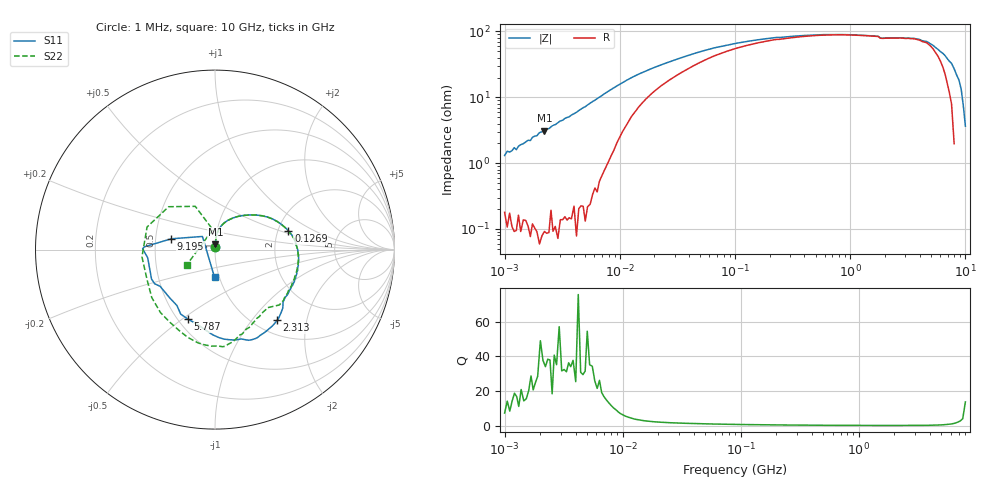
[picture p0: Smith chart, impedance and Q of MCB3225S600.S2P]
!Agilent Technologies,E5071C,MY46111244,A.11.31
!Date: Thu May 09 18:34:08 2019
!Data & Calibration Information:
!Freq	S11:SOLT2(ON)	S21:SOLT2(ON)	S12:SOLT2(ON)	S22:SOLT2(ON)
# Hz S dB R 50
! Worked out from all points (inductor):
!   201 points, 1 MHz to 10 GHz, reference 50 ohm
!   read as one part in series: L = 218 nH near 1.053 MHz
!   highest Q = 37.9 at 2.216 MHz (marker M1), where L = 224 nH
!   self-resonance near 9.967 GHz
!   S11 on the Smith chart (normalised r, x): 1 MHz: 1.00, +0.03; 126.9 MHz: 2.28, +0.58; 2.313 GHz: 1.24, -1.35; 5.787 GHz: 0.56, -0.53; 9.195 GHz: 0.60, +0.08; 10 GHz: 0.95, -0.30
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1000000  -37.49 83.9  -0.00 -0.7  -0.03 -0.7  -37.47 80.1
2216092  -30.49 85.7  -0.01 -1.8  -0.01 -1.9  -30.31 86.1
4810209  -23.33 84.3  -0.05 -4.0  -0.04 -4.1  -23.32 84.8
1.053043e7  -15.96 70.5  -0.37 -9.2  -0.37 -9.2  -15.98 70.6
2.206931e7  -11.82 48.3  -1.39 -13.5  -1.40 -13.5  -11.83 48.3
1.047129e8  -7.72 17.1  -4.08 -14.3  -4.08 -14.3  -7.72 17.0
1.269299e8  -7.49 14.3  -4.34 -13.8  -4.35 -13.8  -7.49 14.1
4.810209e8  -6.62 -4.6  -5.48 -12.4  -5.49 -12.4  -6.64 -5.2
1.380384e9  -6.51 -28.9  -5.72 -21.9  -5.71 -21.9  -6.54 -30.9
2.206931e9  -5.66 -47.1  -5.86 -34.0  -5.84 -34.0  -6.98 -56.3
2.312765e9  -5.61 -48.7  -5.93 -35.4  -5.94 -35.3  -6.97 -58.7
3.801894e9  -5.37 -69.7  -6.53 -51.0  -6.58 -50.9  -5.71 -78.2
4.83488e9  -6.19 -87.5  -6.55 -64.0  -6.54 -64.0  -5.39 -88.1
5.786901e9  -7.62 -111.0  -6.05 -79.5  -6.05 -79.6  -5.54 -100.4
6.952868e9  -8.69 -146.3  -5.19 -101.2  -5.23 -101.4  -6.67 -130.8
7.585776e9  -8.18 -155.1  -4.64 -112.4  -4.64 -112.3  -7.65 -155.6
7.988146e9  -8.46 -173.0  -4.24 -121.1  -4.25 -121.1  -7.77 -174.3
8.390517e9  -7.89 179.3  -3.87 -128.8  -3.87 -128.9  -7.98 161.6
8.792888e9  -8.08 177.8  -2.86 -138.2  -2.90 -138.1  -9.08 137.2
9.195259e9  -12.00 166.1  -1.89 -151.7  -1.98 -151.7  -11.54 114.5
9.597629e9  -19.89 133.7  -1.38 -169.1  -1.39 -169.1  -18.99 96.4
1e10  -16.17 -90.8  -1.36 171.6  -1.34 171.7  -14.88 -151.3
